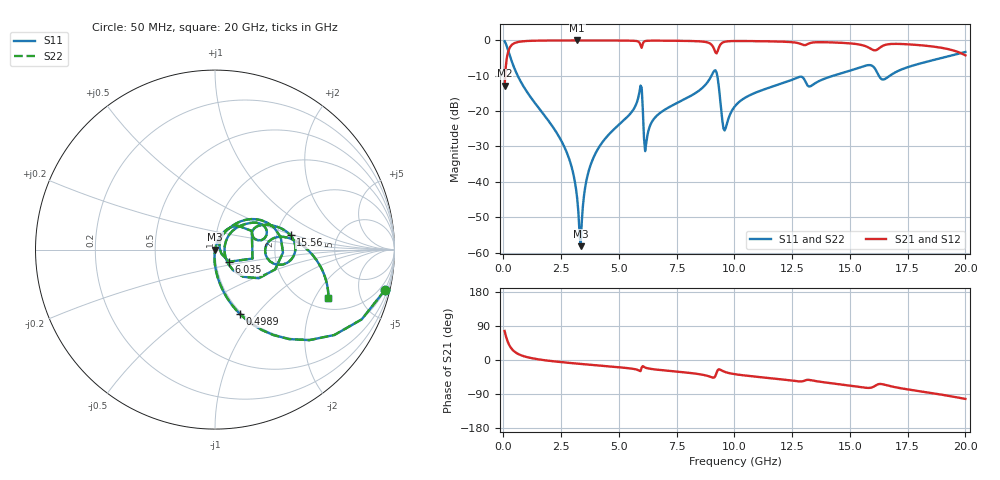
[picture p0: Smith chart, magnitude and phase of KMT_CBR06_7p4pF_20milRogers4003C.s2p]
! Data measured by Modelithics Inc. support@modelithics.com 813-866-6335
! KEMET CBR0603 7.4pF, Pad Width= 0.851mm, Pad Length= 0.64mm, Pad Gap= 0.62mm, 20mil Rogers 4003C substrate Data, January 2022
# hz S ma R 50
! 2 Port Network Data from SP1.SP block
! freq  magS11  angS11  magS21  angS21  magS12  angS12  magS22  angS22
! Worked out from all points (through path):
!   401 points, 50 MHz to 20 GHz, reference 50 ohm
!   highest |S21| = -0.01 dB at 3.192 GHz (marker M1); lowest = -12.8 dB at 50 MHz (marker M2)
!   group delay of S21, straight-line fit = 14.7 ps
!   lowest |S11| = -58.2 dB at 3.342 GHz (marker M3), VSWR 1.00, Z = 50.1 + j0.0243 ohm
!   |S11| at or under -10 dB: 618.6 MHz to 9.005 GHz (8.387 GHz wide, 174 % of centre); 9.256 GHz to 14.27 GHz (5.014 GHz wide, 42.6 % of centre); 16.25 GHz to 16.73 GHz (470.9 MHz wide, 2.86 % of centre)
!   |S22| runs from -58.2 to -0.2 dB; largest |S21 - S12| = 0
!   S11 on the Smith chart (normalised r, x): 50 MHz: 0.98, -8.43; 498.9 MHz: 0.98, -0.83; 6.035 GHz: 1.16, -0.16; 15.56 GHz: 2.39, +0.46; 20 GHz: 2.56, -2.58
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5e7  0.9735 -13.4  0.2283 76.6  0.2283 76.6  0.9735 -13.4
2.495e8  0.6473 -50.4  0.7615 39.6  0.7615 39.6  0.6473 -50.4
4.98875e8  0.3857 -68.8  0.922 21.1  0.922 21.1  0.3857 -68.8
2.6435e9  0.03086 -94.5  0.9984 -6.4  0.9984 -6.4  0.03086 -94.5
2.992625e9  0.01438 -94.1  0.9987 -8.5  0.9987 -8.5  0.01438 -94.1
3.192125e9  0.005829 -88.5  0.9988 -9.6  0.9988 -9.6  0.005829 -88.5
3.34175e9  0.00123 11.4  0.9987 -10.4  0.9987 -10.4  0.00123 11.4
3.391625e9  0.002725 54.3  0.9987 -10.7  0.9987 -10.7  0.002725 54.3
3.641e9  0.01232 72.4  0.9986 -12.0  0.9986 -12.0  0.01232 72.4
4.089875e9  0.02915 73.1  0.9981 -14.3  0.9981 -14.3  0.02915 73.1
5.885375e9  0.1848 46.0  0.9342 -28.4  0.9342 -28.4  0.1848 46.0
6.035e9  0.103 -41.3  0.9056 -16.1  0.9056 -16.1  0.103 -41.3
6.184625e9  0.03583 45.9  0.9852 -21.0  0.9852 -21.0  0.03583 45.9
6.73325e9  0.09169 62.0  0.9925 -26.0  0.9925 -26.0  0.09169 62.0
9.12725e9  0.3727 10.7  0.7461 -46.2  0.7461 -46.2  0.3727 10.7
9.576125e9  0.05327 3.7  0.9555 -31.1  0.9555 -31.1  0.05327 3.7
1.0025e10  0.1176 46.5  0.9804 -37.5  0.9804 -37.5  0.1176 46.5
1.276812e10  0.3019 26.1  0.9143 -56.4  0.9143 -56.4  0.3019 26.1
1.336662e10  0.2322 26.0  0.9323 -53.9  0.9323 -53.9  0.2322 26.0
1.556112e10  0.4281 10.7  0.8525 -72.4  0.8525 -72.4  0.4281 10.7
1.670825e10  0.3135 9.8  0.8869 -68.4  0.8869 -68.4  0.3135 9.8
2e10  0.6862 -22.9  0.6141 -102.6  0.6141 -102.6  0.6862 -22.9
